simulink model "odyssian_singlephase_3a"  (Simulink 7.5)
settings: Solver=ode23t  StartTime=0.0  StopTime=10  RelTol=1e-6
undefined symbols (not defined in the file or in its folder): dfilt, DiscIntNeverNeededParam
libraries: powerlib x61, powerlib_extras x25, simulink x12, dsparch4 x2
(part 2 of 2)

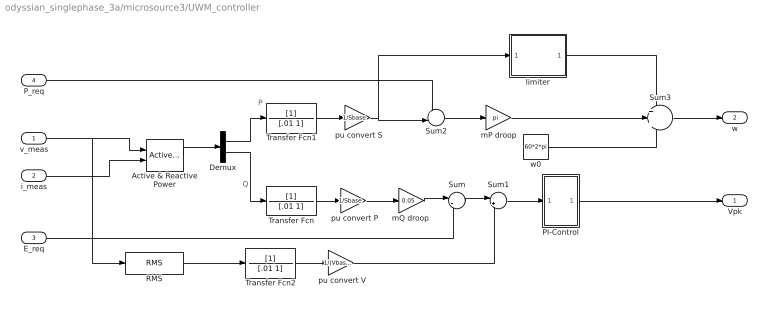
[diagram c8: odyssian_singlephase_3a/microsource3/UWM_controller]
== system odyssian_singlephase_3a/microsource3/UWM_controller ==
  note: P
  note: Q
  v_meas : Inport
  i_meas : Inport  Port=2
  E_req : Inport  Port=3
  P_req : Inport  Port=4
  " pu convert P" : Gain  Gain=1/Sbase  ParameterDataType=sfix(16)  ParameterScaling=2^0  OutDataType=sfix(16)  OutScaling=2^0
  " pu convert S" : Gain  Gain=1/Sbase  ParameterDataType=sfix(16)  ParameterScaling=2^0  OutDataType=sfix(16)  OutScaling=2^0
  " pu convert V" : Gain  Gain=1/(Vbase/sqrt(2))  ParameterDataType=sfix(16)  ParameterScaling=2^0  OutDataType=sfix(16)  OutScaling=2^0
  Active & Reactive Power : powerlib_extras/Measurements/Active & Reactive Power  DialogController=POWERSYS.PowerSysDialog  SystemSampleTime=-1  f1=60
  Demux : Demux  Outputs=2
  PI-Control : Subsystem
  RMS : powerlib_extras/Measurements/RMS  DialogController=POWERSYS.PowerSysDialog  SystemSampleTime=-1  f1=60
  Sum : Sum  Inputs=|-+  OutDataType=sfix(16)  OutScaling=2^0
  Sum1 : Sum  Inputs=|+-  OutDataType=sfix(16)  OutScaling=2^0
  Sum2 : Sum  Inputs=+-|  OutDataType=sfix(16)  OutScaling=2^0
  Sum3 : Sum  Inputs=+++  OutDataType=sfix(16)  OutScaling=2^0
  Transfer Fcn : TransferFcn  Denominator=[.01 1]
  Transfer Fcn1 : TransferFcn  Denominator=[.01 1]
  Transfer Fcn2 : TransferFcn  Denominator=[.01 1]
  limiter : Subsystem
  mP droop : Gain  Gain=pi  ParameterDataType=sfix(16)  ParameterScaling=2^0  OutDataType=sfix(16)  OutScaling=2^0
  "mQ droop " : Gain  Gain=0.05  ParameterDataType=sfix(16)  ParameterScaling=2^0  OutDataType=sfix(16)  OutScaling=2^0
  w0 : Constant  Value=60*2*pi  OutDataType=fixdt(1, 16)  OutScaling=2^0
  Vpk : Outport
  w : Outport  Port=2
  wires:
  Transfer Fcn2/1 -> " pu convert V"/1
  Transfer Fcn/1 -> " pu convert P"/1
  " pu convert P"/1 -> "mQ droop "/1
  Transfer Fcn1/1 -> " pu convert S"/1
  " pu convert S"/1 -> limiter/1(In1), Sum2/2
  i_meas/1 -> Active & Reactive Power/2
  P_req/1 -> Sum2/1
  mP droop/1 -> Sum3/2
  limiter/1(Out1) -> Sum3/1
  w0/1 -> Sum3/3
  Sum2/1 -> mP droop/1
  Sum1/1 -> PI-Control/1(In1)
  Sum/1 -> Sum1/1
  "mQ droop "/1 -> Sum/1
  Demux/2 -> Transfer Fcn/1
  Demux/1 -> Transfer Fcn1/1
  Active & Reactive Power/1 -> Demux/1
  v_meas/1 -> RMS/1, Active & Reactive Power/1
  PI-Control/1(Out1) -> Vpk/1
  Sum3/1 -> w/1
  E_req/1 -> Sum/2
  " pu convert V"/1 -> Sum1/2
  RMS/1 -> Transfer Fcn2/1

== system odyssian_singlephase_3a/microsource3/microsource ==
  Vpk : Inport  OutDataType=fixdt(1, 16)  OutScaling=2^0
  w : Inport  Port=2  OutDataType=fixdt(1, 16)  OutScaling=2^0
  Integrator : Integrator
  Product : Product  OutDataType=sfix(16)  OutScaling=2^0
  phaseA : powerlib/Electrical Sources/Controlled Voltage Source  DialogController=POWERSYS.PowerSysDialog  SystemSampleTime=-1  Initialize=on  Source_Type=AC  Amplitude=0  Phase=0  Frequency=0  Measurements=None
  v_A : Fcn  Expr=cos(u)
  Va : PMIOPort  Tag=PMCPort  Port=1  Side=Right
  Neutral : PMIOPort  Tag=PMCPort  Port=2  Side=Right
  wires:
  Product/1 -> phaseA/1
  Vpk/1 -> Product/1
  w/1 -> Integrator/1
  Integrator/1 -> v_A/1
  v_A/1 -> Product/2
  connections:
  phaseA/RConn1 -- Va/RConn1
  phaseA/LConn1 -- Neutral/RConn1

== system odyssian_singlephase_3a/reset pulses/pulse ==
  Step : Step  Time=tstart  SampleTime=0
  Step1 : Step  Time=tstart+dt  After=-1  SampleTime=0
  Sum : Sum  Inputs=|++  OutDataType=fixdt(1, 16)  OutScaling=2^0
  Out1 : Outport
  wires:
  Step/1 -> Sum/2
  Step1/1 -> Sum/1
  Sum/1 -> Out1/1

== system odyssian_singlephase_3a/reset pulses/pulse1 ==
  Step : Step  Time=tstart  SampleTime=0
  Step1 : Step  Time=tstart+dt  After=-1  SampleTime=0
  Sum : Sum  Inputs=|++  OutDataType=fixdt(1, 16)  OutScaling=2^0
  Out1 : Outport
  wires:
  Step/1 -> Sum/2
  Step1/1 -> Sum/1
  Sum/1 -> Out1/1

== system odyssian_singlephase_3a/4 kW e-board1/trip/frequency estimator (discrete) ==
  v : Inport
  Constant : Constant  Value=60  OutDataType=fixdt(1, 16)  OutScaling=2^0
  Fcn : Fcn  Expr=sin(2*pi*u[1])
  Filter Quantized : Subsystem  Tag=BlockMethodSubSystem
  Gain : Gain  Gain=1/150  ParameterDataType=fixdt(1, 16)  ParameterScaling=2^0  OutDataType=fixdt(1, 16)  OutScaling=2^0  SampleTime=dt
  Product : Product  OutDataType=fixdt(1, 16)  OutScaling=2^0
  Scope : Scope
  Sum : Sum  Inputs=|++  OutDataType=fixdt(1, 16)  OutScaling=2^0
  modulo discrete integrator : Subsystem  mask{dt=dt}
      mask prompts: dt "sample time"
  w : Outport  OutDataType=fixdt(1, 16)  OutScaling=2^0
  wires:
  Fcn/1 -> Product/2
  Constant/1 -> Sum/2
  modulo discrete integrator/1(Out1) -> Fcn/1
  Sum/1 -> modulo discrete integrator/1(In1), w/1
  Product/1 -> Filter Quantized/1(In)
  Filter Quantized/1(Out) -> Scope/1, Sum/1
  v/1 -> Gain/1
  Gain/1 -> Product/1

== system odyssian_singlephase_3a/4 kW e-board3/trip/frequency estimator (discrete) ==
  v : Inport
  Constant : Constant  Value=60  OutDataType=fixdt(1, 16)  OutScaling=2^0
  Fcn : Fcn  Expr=sin(2*pi*u[1])
  Filter Quantized : Subsystem  Tag=BlockMethodSubSystem
  Gain : Gain  Gain=1/150  ParameterDataType=fixdt(1, 16)  ParameterScaling=2^0  OutDataType=fixdt(1, 16)  OutScaling=2^0  SampleTime=dt
  Product : Product  OutDataType=fixdt(1, 16)  OutScaling=2^0
  Scope : Scope
  Sum : Sum  Inputs=|++  OutDataType=fixdt(1, 16)  OutScaling=2^0
  modulo discrete integrator : Subsystem  mask{dt=dt}
      mask prompts: dt "sample time"
  w : Outport  OutDataType=fixdt(1, 16)  OutScaling=2^0
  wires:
  Fcn/1 -> Product/2
  Constant/1 -> Sum/2
  modulo discrete integrator/1(Out1) -> Fcn/1
  Sum/1 -> modulo discrete integrator/1(In1), w/1
  Product/1 -> Filter Quantized/1(In)
  Filter Quantized/1(Out) -> Scope/1, Sum/1
  v/1 -> Gain/1
  Gain/1 -> Product/1

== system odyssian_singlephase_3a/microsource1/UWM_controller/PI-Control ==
  In1 : Inport
  Gain : Gain  Gain=.01  ParameterDataType=sfix(16)  ParameterScaling=2^0  OutDataType=sfix(16)  OutScaling=2^0
  Gain1 : Gain  Gain=5  ParameterDataType=sfix(16)  ParameterScaling=2^0  OutDataType=sfix(16)  OutScaling=2^0
  Gain2 : Gain  Gain=750  ParameterDataType=sfix(16)  ParameterScaling=2^0  OutDataType=sfix(16)  OutScaling=2^0
  Integrator1 : Integrator  LimitOutput=on  UpperSaturationLimit=100  LowerSaturationLimit=-100  ZeroCross=off
  Sum4 : Sum  Inputs=|++  OutDataType=sfix(16)  OutScaling=2^0
  Out1 : Outport
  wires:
  Gain/1 -> Sum4/1
  Integrator1/1 -> Sum4/2
  In1/1 -> Gain1/1, Gain/1
  Gain1/1 -> Integrator1/1
  Sum4/1 -> Gain2/1
  Gain2/1 -> Out1/1

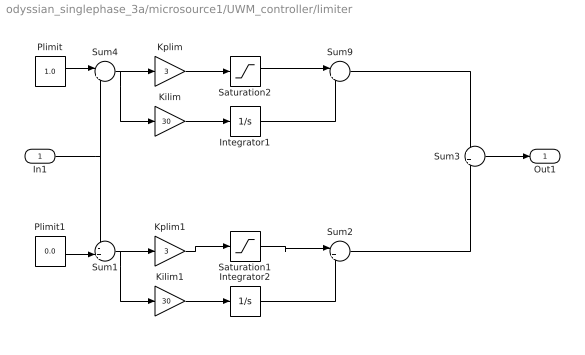
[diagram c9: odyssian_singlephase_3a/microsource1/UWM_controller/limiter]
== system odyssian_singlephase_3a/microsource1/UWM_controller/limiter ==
  In1 : Inport
  Integrator1 : Integrator  LimitOutput=on  UpperSaturationLimit=0  LowerSaturationLimit=-pi  ZeroCross=off
  Integrator2 : Integrator  LimitOutput=on  UpperSaturationLimit=pi  LowerSaturationLimit=0  ZeroCross=off
  Kilim : Gain  Gain=30  ParameterDataType=sfix(16)  ParameterScaling=2^0  OutDataType=sfix(16)  OutScaling=2^0
  Kilim1 : Gain  Gain=30  ParameterDataType=sfix(16)  ParameterScaling=2^0  OutDataType=sfix(16)  OutScaling=2^0
  Kplim : Gain  Gain=3  ParameterDataType=sfix(16)  ParameterScaling=2^0  OutDataType=sfix(16)  OutScaling=2^0
  Kplim1 : Gain  Gain=3  ParameterDataType=sfix(16)  ParameterScaling=2^0  OutDataType=sfix(16)  OutScaling=2^0
  Plimit : Constant  Value=1.0  OutDataType=sfix(16)  OutScaling=2^0
  Plimit1 : Constant  Value=0.0  OutDataType=sfix(16)  OutScaling=2^0
  Saturation1 : Saturate  UpperLimit=pi  LowerLimit=0  OutDataType=fixdt(1, 16)  OutScaling=2^0
  Saturation2 : Saturate  UpperLimit=0  LowerLimit=-pi  OutDataType=fixdt(1, 16)  OutScaling=2^0
  Sum1 : Sum  Inputs=-+|  OutDataType=sfix(16)  OutScaling=2^0
  Sum2 : Sum  Inputs=|++  OutDataType=sfix(16)  OutScaling=2^0
  Sum3 : Sum  OutDataType=sfix(16)  OutScaling=2^0
  Sum4 : Sum  Inputs=|+-  OutDataType=sfix(16)  OutScaling=2^0
  Sum9 : Sum  Inputs=|++  OutDataType=sfix(16)  OutScaling=2^0
  Out1 : Outport
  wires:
  Sum3/1 -> Out1/1
  Plimit1/1 -> Sum1/2
  Integrator2/1 -> Sum2/2
  Kilim1/1 -> Integrator2/1
  Sum1/1 -> Kilim1/1, Kplim1/1
  In1/1 -> Sum1/1, Sum4/2
  Integrator1/1 -> Sum9/2
  Kilim/1 -> Integrator1/1
  Sum4/1 -> Kilim/1, Kplim/1
  Plimit/1 -> Sum4/1
  Kplim1/1 -> Saturation1/1
  Saturation1/1 -> Sum2/1
  Kplim/1 -> Saturation2/1
  Saturation2/1 -> Sum9/1
  Sum9/1 -> Sum3/1
  Sum2/1 -> Sum3/2

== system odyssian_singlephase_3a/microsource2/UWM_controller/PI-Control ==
  In1 : Inport
  Gain : Gain  Gain=.01  ParameterDataType=sfix(16)  ParameterScaling=2^0  OutDataType=sfix(16)  OutScaling=2^0
  Gain1 : Gain  Gain=5  ParameterDataType=sfix(16)  ParameterScaling=2^0  OutDataType=sfix(16)  OutScaling=2^0
  Gain2 : Gain  Gain=750  ParameterDataType=sfix(16)  ParameterScaling=2^0  OutDataType=sfix(16)  OutScaling=2^0
  Integrator1 : Integrator  LimitOutput=on  UpperSaturationLimit=100  LowerSaturationLimit=-100  ZeroCross=off
  Sum4 : Sum  Inputs=|++  OutDataType=sfix(16)  OutScaling=2^0
  Out1 : Outport
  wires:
  Gain/1 -> Sum4/1
  Integrator1/1 -> Sum4/2
  In1/1 -> Gain1/1, Gain/1
  Gain1/1 -> Integrator1/1
  Sum4/1 -> Gain2/1
  Gain2/1 -> Out1/1

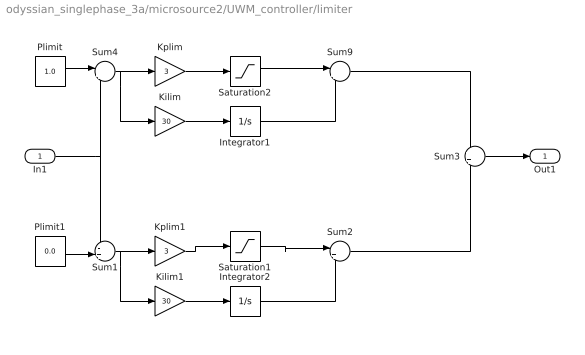
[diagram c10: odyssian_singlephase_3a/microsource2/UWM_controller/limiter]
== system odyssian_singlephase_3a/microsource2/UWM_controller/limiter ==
  In1 : Inport
  Integrator1 : Integrator  LimitOutput=on  UpperSaturationLimit=0  LowerSaturationLimit=-pi  ZeroCross=off
  Integrator2 : Integrator  LimitOutput=on  UpperSaturationLimit=pi  LowerSaturationLimit=0  ZeroCross=off
  Kilim : Gain  Gain=30  ParameterDataType=sfix(16)  ParameterScaling=2^0  OutDataType=sfix(16)  OutScaling=2^0
  Kilim1 : Gain  Gain=30  ParameterDataType=sfix(16)  ParameterScaling=2^0  OutDataType=sfix(16)  OutScaling=2^0
  Kplim : Gain  Gain=3  ParameterDataType=sfix(16)  ParameterScaling=2^0  OutDataType=sfix(16)  OutScaling=2^0
  Kplim1 : Gain  Gain=3  ParameterDataType=sfix(16)  ParameterScaling=2^0  OutDataType=sfix(16)  OutScaling=2^0
  Plimit : Constant  Value=1.0  OutDataType=sfix(16)  OutScaling=2^0
  Plimit1 : Constant  Value=0.0  OutDataType=sfix(16)  OutScaling=2^0
  Saturation1 : Saturate  UpperLimit=pi  LowerLimit=0  OutDataType=fixdt(1, 16)  OutScaling=2^0
  Saturation2 : Saturate  UpperLimit=0  LowerLimit=-pi  OutDataType=fixdt(1, 16)  OutScaling=2^0
  Sum1 : Sum  Inputs=-+|  OutDataType=sfix(16)  OutScaling=2^0
  Sum2 : Sum  Inputs=|++  OutDataType=sfix(16)  OutScaling=2^0
  Sum3 : Sum  OutDataType=sfix(16)  OutScaling=2^0
  Sum4 : Sum  Inputs=|+-  OutDataType=sfix(16)  OutScaling=2^0
  Sum9 : Sum  Inputs=|++  OutDataType=sfix(16)  OutScaling=2^0
  Out1 : Outport
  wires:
  Sum3/1 -> Out1/1
  Plimit1/1 -> Sum1/2
  Integrator2/1 -> Sum2/2
  Kilim1/1 -> Integrator2/1
  Sum1/1 -> Kilim1/1, Kplim1/1
  In1/1 -> Sum1/1, Sum4/2
  Integrator1/1 -> Sum9/2
  Kilim/1 -> Integrator1/1
  Sum4/1 -> Kilim/1, Kplim/1
  Plimit/1 -> Sum4/1
  Kplim1/1 -> Saturation1/1
  Saturation1/1 -> Sum2/1
  Kplim/1 -> Saturation2/1
  Saturation2/1 -> Sum9/1
  Sum9/1 -> Sum3/1
  Sum2/1 -> Sum3/2

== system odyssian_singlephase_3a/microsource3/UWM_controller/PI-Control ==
  In1 : Inport
  Gain : Gain  Gain=.01  ParameterDataType=sfix(16)  ParameterScaling=2^0  OutDataType=sfix(16)  OutScaling=2^0
  Gain1 : Gain  Gain=5  ParameterDataType=sfix(16)  ParameterScaling=2^0  OutDataType=sfix(16)  OutScaling=2^0
  Gain2 : Gain  Gain=750  ParameterDataType=sfix(16)  ParameterScaling=2^0  OutDataType=sfix(16)  OutScaling=2^0
  Integrator1 : Integrator  LimitOutput=on  UpperSaturationLimit=100  LowerSaturationLimit=-100  ZeroCross=off
  Sum4 : Sum  Inputs=|++  OutDataType=sfix(16)  OutScaling=2^0
  Out1 : Outport
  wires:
  Gain/1 -> Sum4/1
  Integrator1/1 -> Sum4/2
  In1/1 -> Gain1/1, Gain/1
  Gain1/1 -> Integrator1/1
  Sum4/1 -> Gain2/1
  Gain2/1 -> Out1/1

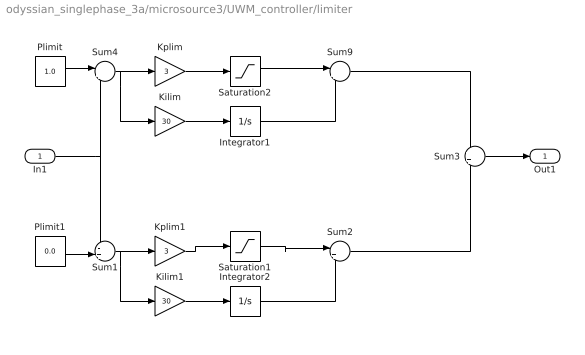
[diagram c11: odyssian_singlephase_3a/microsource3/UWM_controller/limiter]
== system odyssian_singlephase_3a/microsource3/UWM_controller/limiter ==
  In1 : Inport
  Integrator1 : Integrator  LimitOutput=on  UpperSaturationLimit=0  LowerSaturationLimit=-pi  ZeroCross=off
  Integrator2 : Integrator  LimitOutput=on  UpperSaturationLimit=pi  LowerSaturationLimit=0  ZeroCross=off
  Kilim : Gain  Gain=30  ParameterDataType=sfix(16)  ParameterScaling=2^0  OutDataType=sfix(16)  OutScaling=2^0
  Kilim1 : Gain  Gain=30  ParameterDataType=sfix(16)  ParameterScaling=2^0  OutDataType=sfix(16)  OutScaling=2^0
  Kplim : Gain  Gain=3  ParameterDataType=sfix(16)  ParameterScaling=2^0  OutDataType=sfix(16)  OutScaling=2^0
  Kplim1 : Gain  Gain=3  ParameterDataType=sfix(16)  ParameterScaling=2^0  OutDataType=sfix(16)  OutScaling=2^0
  Plimit : Constant  Value=1.0  OutDataType=sfix(16)  OutScaling=2^0
  Plimit1 : Constant  Value=0.0  OutDataType=sfix(16)  OutScaling=2^0
  Saturation1 : Saturate  UpperLimit=pi  LowerLimit=0  OutDataType=fixdt(1, 16)  OutScaling=2^0
  Saturation2 : Saturate  UpperLimit=0  LowerLimit=-pi  OutDataType=fixdt(1, 16)  OutScaling=2^0
  Sum1 : Sum  Inputs=-+|  OutDataType=sfix(16)  OutScaling=2^0
  Sum2 : Sum  Inputs=|++  OutDataType=sfix(16)  OutScaling=2^0
  Sum3 : Sum  OutDataType=sfix(16)  OutScaling=2^0
  Sum4 : Sum  Inputs=|+-  OutDataType=sfix(16)  OutScaling=2^0
  Sum9 : Sum  Inputs=|++  OutDataType=sfix(16)  OutScaling=2^0
  Out1 : Outport
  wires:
  Sum3/1 -> Out1/1
  Plimit1/1 -> Sum1/2
  Integrator2/1 -> Sum2/2
  Kilim1/1 -> Integrator2/1
  Sum1/1 -> Kilim1/1, Kplim1/1
  In1/1 -> Sum1/1, Sum4/2
  Integrator1/1 -> Sum9/2
  Kilim/1 -> Integrator1/1
  Sum4/1 -> Kilim/1, Kplim/1
  Plimit/1 -> Sum4/1
  Kplim1/1 -> Saturation1/1
  Saturation1/1 -> Sum2/1
  Kplim/1 -> Saturation2/1
  Saturation2/1 -> Sum9/1
  Sum9/1 -> Sum3/1
  Sum2/1 -> Sum3/2

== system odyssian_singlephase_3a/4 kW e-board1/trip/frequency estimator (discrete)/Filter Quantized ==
  In : Inport
  Input Quantizer : DataTypeConversion  OutDataTypeMode=Specify via dialog  OutDataType=fixdt(1,16,15)  OutDataTypeStr=fixdt(1,16,15)  RndMeth=Round
  filter : dsparch4/Biquad Filter  DialogController=dspdialog.BiquadFilter  DialogControllerArgs=DataTag0  IIRFiltStruct=Direct form II  CoeffSource=Specify via dialog  BiQuadCoeffs=[1 -1.35890654546667 1 1 -1.77683423091592 0.868775728611993;1 1 0 1 -0.84680556917748 0]  a0Flag=Warning  IC=0  ICnum=0  ICden=0  firstCoeffMode=Binary point scaling  firstCoeffWordLength=16  firstCoeffFracLength=14  outputMode=Binary point scaling  outputWordLength=16  outputFracLength=11  accumMode=Binary point scaling  accumWordLength=40  accumFracLength=29  denAccumFracLength=29  prodOutputMode=Binary point scaling  prodOutputWordLength=32  prodOutputFracLength=29  denProdOutputFracLength=29  memoryMode=Binary point scaling  memoryWordLength=16  memoryFracLength=15  secondMemoryFracLength=15  roundingMode=Convergent  overflowMode=off  ScaleValues=[0.0483208011510974;0.227336456672284;1]  optimizeScaleValues=on  ScaleValueMode=Specify via input port (g)  scaleValueFracLength=17  stageInputMode=Binary point scaling  stageOutputMode=Binary point scaling  stageInputWordLength=16  stageInputFracLength=12  stageOutputWordLength=16  stageOutputFracLength=11  FilterSource=Specify via dialog  dfiltObjectName=dfilt.df2tsos([1 0.3 0.4],[1 0.1 0.2])
  Out : Outport
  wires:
  In/1 -> Input Quantizer/1
  Input Quantizer/1 -> filter/1
  filter/1 -> Out/1

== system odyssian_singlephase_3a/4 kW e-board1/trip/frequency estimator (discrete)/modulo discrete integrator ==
  In1 : Inport
  Abs : Abs
  Constant1 : Constant  OutDataType=sfix(16)  OutScaling=2^0
  Discrete-Time Integrator : DiscreteIntegrator  ExternalReset=rising  InitialConditionSource=external  SampleTime=dt  OutDataType=fixdt(1, 16)  OutScaling=2^0  UpperSaturationLimit=100  LowerSaturationLimit=-100  ShowStatePort=on  ICPrevOutput=DiscIntNeverNeededParam  ICPrevScaledInput=DiscIntNeverNeededParam
  Gain1 : Gain  Gain=1+.0001  ParameterDataType=sfix(16)  ParameterScaling=2^0  OutDataType=sfix(16)  OutScaling=2^0
  IC : InitialCondition  Value=0
  Math Function : Math  Operator=rem  OutDataType=sfix(16)  OutScaling=2^0
  Relational Operator : RelationalOperator
  Out1 : Outport
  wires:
  Relational Operator/1 -> Discrete-Time Integrator/2
  Discrete-Time Integrator/State -> Gain1/1
  Gain1/1 -> Abs/1
  Constant1/1 -> Relational Operator/2, Math Function/2
  Abs/1 -> Relational Operator/1, Math Function/1
  In1/1 -> Discrete-Time Integrator/1
  Discrete-Time Integrator/1 -> Out1/1
  IC/1 -> Discrete-Time Integrator/3
  Math Function/1 -> IC/1

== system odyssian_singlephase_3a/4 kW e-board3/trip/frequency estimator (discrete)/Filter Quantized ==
  In : Inport
  Input Quantizer : DataTypeConversion  OutDataTypeMode=Specify via dialog  OutDataType=fixdt(1,16,15)  OutDataTypeStr=fixdt(1,16,15)  RndMeth=Round
  filter : dsparch4/Biquad Filter  DialogController=dspdialog.BiquadFilter  DialogControllerArgs=DataTag1  IIRFiltStruct=Direct form II  CoeffSource=Specify via dialog  BiQuadCoeffs=[1 -1.35890654546667 1 1 -1.77683423091592 0.868775728611993;1 1 0 1 -0.84680556917748 0]  a0Flag=Warning  IC=0  ICnum=0  ICden=0  firstCoeffMode=Binary point scaling  firstCoeffWordLength=16  firstCoeffFracLength=14  outputMode=Binary point scaling  outputWordLength=16  outputFracLength=11  accumMode=Binary point scaling  accumWordLength=40  accumFracLength=29  denAccumFracLength=29  prodOutputMode=Binary point scaling  prodOutputWordLength=32  prodOutputFracLength=29  denProdOutputFracLength=29  memoryMode=Binary point scaling  memoryWordLength=16  memoryFracLength=15  secondMemoryFracLength=15  roundingMode=Convergent  overflowMode=off  ScaleValues=[0.0483208011510974;0.227336456672284;1]  optimizeScaleValues=on  ScaleValueMode=Specify via input port (g)  scaleValueFracLength=17  stageInputMode=Binary point scaling  stageOutputMode=Binary point scaling  stageInputWordLength=16  stageInputFracLength=12  stageOutputWordLength=16  stageOutputFracLength=11  FilterSource=Specify via dialog  dfiltObjectName=dfilt.df2tsos([1 0.3 0.4],[1 0.1 0.2])
  Out : Outport
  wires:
  In/1 -> Input Quantizer/1
  Input Quantizer/1 -> filter/1
  filter/1 -> Out/1

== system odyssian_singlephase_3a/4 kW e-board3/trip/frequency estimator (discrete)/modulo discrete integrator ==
  In1 : Inport
  Abs : Abs
  Constant1 : Constant  OutDataType=sfix(16)  OutScaling=2^0
  Discrete-Time Integrator : DiscreteIntegrator  ExternalReset=rising  InitialConditionSource=external  SampleTime=dt  OutDataType=fixdt(1, 16)  OutScaling=2^0  UpperSaturationLimit=100  LowerSaturationLimit=-100  ShowStatePort=on  ICPrevOutput=DiscIntNeverNeededParam  ICPrevScaledInput=DiscIntNeverNeededParam
  Gain1 : Gain  Gain=1+.0001  ParameterDataType=sfix(16)  ParameterScaling=2^0  OutDataType=sfix(16)  OutScaling=2^0
  IC : InitialCondition  Value=0
  Math Function : Math  Operator=rem  OutDataType=sfix(16)  OutScaling=2^0
  Relational Operator : RelationalOperator
  Out1 : Outport
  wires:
  Relational Operator/1 -> Discrete-Time Integrator/2
  Discrete-Time Integrator/State -> Gain1/1
  Gain1/1 -> Abs/1
  Constant1/1 -> Relational Operator/2, Math Function/2
  Abs/1 -> Relational Operator/1, Math Function/1
  In1/1 -> Discrete-Time Integrator/1
  Discrete-Time Integrator/1 -> Out1/1
  IC/1 -> Discrete-Time Integrator/3
  Math Function/1 -> IC/1
